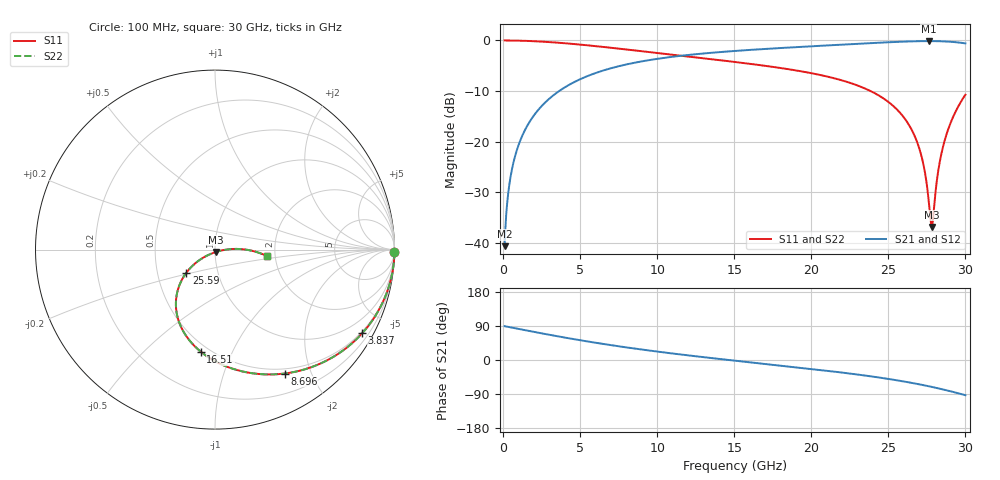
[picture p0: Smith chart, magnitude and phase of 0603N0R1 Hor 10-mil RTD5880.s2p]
# GHz S MA R 50
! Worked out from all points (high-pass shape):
!   3201 points, 100 MHz to 30 GHz, reference 50 ohm
!   highest |S21| = -0.13 dB at 27.62 GHz (marker M1); lowest = -40.7 dB at 100 MHz (marker M2)
!   |S21| within 3 dB of the highest: 11.27 GHz to end of sweep
!   lowest |S11| = -36.9 dB at 27.81 GHz (marker M3), VSWR 1.03, Z = 50.4 - j1.38 ohm
!   |S11| at or under -10 dB: 23.84 GHz to end of sweep
!   |S22| runs from -36.9 to 0.0 dB; largest |S21 - S12| = 0
!   S11 on the Smith chart (normalised r, x): 100 MHz: open; 3.837 GHz: 0.44, -3.74; 8.696 GHz: 0.44, -1.62; 16.51 GHz: 0.45, -0.76; 25.59 GHz: 0.70, -0.19; 30 GHz: 1.80, -0.14
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0.1  1 -0.8  0.009243 89.2  0.009243 89.2  1 -0.8
0.4924375  0.999 -3.9  0.04546 86.1  0.04546 86.1  0.999 -3.9
1.118469  0.9947 -8.9  0.1027 81.1  0.1027 81.1  0.9947 -8.9
2.211688  0.9798 -17.4  0.1996 72.6  0.1996 72.6  0.9798 -17.4
3.8375  0.9434 -29.6  0.3312 60.4  0.3312 60.4  0.9434 -29.6
5.089563  0.9074 -38.4  0.4195 51.6  0.4195 51.6  0.9074 -38.4
8.69625  0.7922 -60.6  0.609 29.3  0.609 29.3  0.7922 -60.6
10.06978  0.7498 -68.0  0.6601 21.9  0.6601 21.9  0.7498 -68.0
15.05  0.6125 -91.5  0.7878 -1.8  0.7878 -1.8  0.6125 -91.5
16.50763  0.5745 -97.9  0.8153 -8.2  0.8153 -8.2  0.5745 -97.9
20.03956  0.4735 -113.3  0.8761 -23.8  0.8761 -23.8  0.4735 -113.3
25.01978  0.2455 -138.0  0.9601 -50.1  0.9601 -50.1  0.2455 -138.0
25.58975  0.2055 -141.1  0.9685 -53.8  0.9685 -53.8  0.2055 -141.1
26.93525  0.09249 -146.0  0.9831 -63.6  0.9831 -63.6  0.09249 -146.0
27.32769  0.05433 -142.8  0.9851 -66.8  0.9851 -66.8  0.05433 -142.8
27.61734  0.02606 -127.2  0.9856 -69.2  0.9856 -69.2  0.02606 -127.2
27.81356  0.01428 -72.7  0.9853 -70.9  0.9853 -70.9  0.01428 -72.7
27.92569  0.01904 -31.8  0.985 -71.9  0.985 -71.9  0.01904 -31.8
28.28075  0.05635 -1.1  0.9827 -75.1  0.9827 -75.1  0.05635 -1.1
28.63581  0.09994 2.0  0.9783 -78.5  0.9783 -78.5  0.09994 2.0
29.24316  0.181 -0.5  0.965 -84.7  0.965 -84.7  0.181 -0.5
30  0.2907 -7.0  0.9359 -92.9  0.9359 -92.9  0.2907 -7.0
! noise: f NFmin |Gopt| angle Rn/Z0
0.1  0.001377  0.9908  0.7841  0.03432
3.417  0.003099  0.7944  14.95  0.003061
6.743  0.004958  0.7304  23.04  0.003521
10.06  0.006863  0.7055  30.85  0.004261
13.39  0.008985  0.699  38.62  0.005221
16.7  0.01151  0.7051  46.25  0.006515
20.03  0.01473  0.7217  53.76  0.008403
23.35  0.01913  0.7476  61.12  0.01139
26.67  0.02572  0.7828  68.43  0.01673
30  0.03683  0.8268  75.75  0.02802
